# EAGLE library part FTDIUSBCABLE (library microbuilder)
FTDI TTL-232R USB Cable Connector for FTDI's USB->RS232 Cable
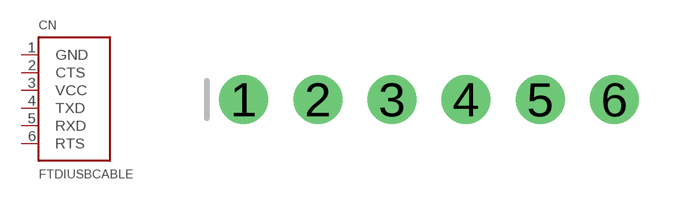
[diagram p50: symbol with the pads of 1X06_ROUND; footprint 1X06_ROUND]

Designator prefix CN

## FTDIUSBCABLE  [1X06_ROUND]
1  GND
2  CTS
3  VCC
4  TXD
5  RXD
6  RTS

## Footprint 1X06_ROUND (pad centres in mm)
PIN HEADER
drill 1 pad 1.676: 1 -6.35,0; 2 -3.81,0; 3 -1.27,0; 4 1.27,0; 5 3.81,0; 6 6.35,0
